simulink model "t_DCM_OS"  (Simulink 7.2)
settings: Solver=ode3  SolverMode=SingleTasking  StartTime=0.0  StopTime=1  FixedStep=10e-6  RelTol=1e-5  AbsTol=1e-6
libraries: simulink x1

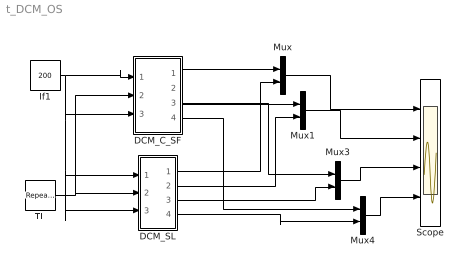
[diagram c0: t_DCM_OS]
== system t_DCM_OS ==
  DCM_C_SF : Subsystem  mask(DCM C-S-Function Block
){Ra=.5, La=3e-3, Rf=200, Lf=1, If0=1, Laf=0.7, J=.0167, D=0.01, W0=0}
      mask prompts: Ra "Armature Resistance"; La "Armature Inductance"; Rf "Field Resistance"; Lf "Filed Inductance"; If0 "Initial field current"; Laf "Mutual Inductance"; J "Moment of Inertia"; D "Damping Coefficient"; W0 "initial ang. speed"
      mask help: Open source D-Motor modeled as Simulink C-S-Function Block Input Vector u: u[0]= Armature Voltage u[1]= Load Torque u[2]= Field Voltage Output Vector y: y[0]= Armature Current y[1]= EMF y[2]= Te y[3]= Ang. Velocity W Parameter Vector p: p[0]= Armature Resistance Ra p[1]= Armature Inductance La p[2]= Field Resistance Rf p[3]= Filed Inductance Lf p[4]= Initial field current ILf0 p[5]= Mutual Ind. Laf p[6]= Moment of Inertia J p[7]= Damp. Coef. D p[8]= Initial Ang. Velocity W0 You can pause the simulation during running, change the Parameters you want and continue the Simulation
  DCM_SL : Subsystem  mask(dcm){Ra=.5, La=3e-3, Rf=200, Lf=1, If0=1, Laf=0.7, J=.0167, D=0.01, omm0=0}
      mask prompts: Ra "Armature Resistance"; La "Armature Inductance"; Rf "Filed Resistance"; Lf "Filed Inductance"; If0 "Initial field current"; Laf "Mutual Inductance"; J "Moment of Inertia"; D "Damping Coefficient"; omm0 "initial ang. speed"
      mask help: Open source D-Motor modeled in Simulink Blocks Input Vector u: u[0]= Armature Voltage u[1]= Load Torque u[2]= Field Voltage Output Vector y: y[0]= Armature Current y[1]= EMF y[2]= Te y[3]= Ang. Velocity W Parameter Vector p: p[0]= Armature Resistance Ra p[1]= Armature Inductance La p[2]= Field Resistance Rf p[3]= Filed Inductance Lf p[4]= Initial field current ILf0 p[5]= Mutual Ind. Laf p[6]= Moment of Inertia J p[7]= Damp. Coef. D p[8]= Initial Ang. Velocity W0 You can pause the simulation during running, change the Parameters you want and continue the Simulation
  If1 : Constant  Value=200
  Mux{,1,3..4} (4 alike) : Mux  Inputs=2
  Scope : Scope  NumInputPorts=4
  TL : simulink/Sources/Repeating Sequence  SystemSampleTime=-1  rep_seq_t="[0   0.2   0.201    0.6    0.601      2 ]"  rep_seq_y="[0     0        40      40      -40      -40]"
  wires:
  DCM_SL/1(ia) -> Mux/2
  DCM_SL/2(emf) -> Mux1/2
  Mux/1 -> Scope/1
  Mux1/1 -> Scope/2
  Mux3/1 -> Scope/3
  DCM_SL/3(Te) -> Mux3/2
  DCM_SL/4(w) -> Mux4/2
  Mux4/1 -> Scope/4
  If1/1 -> DCM_SL/3(Vf), DCM_SL/1(Va), DCM_C_SF/3(vf), DCM_C_SF/1(va)
  TL/1 -> DCM_SL/2(Tl), DCM_C_SF/2(TL)
  DCM_C_SF/1(Ia) -> Mux/1
  DCM_C_SF/2(emf) -> Mux1/1
  DCM_C_SF/3(TE) -> Mux3/1
  DCM_C_SF/4(W) -> Mux4/1

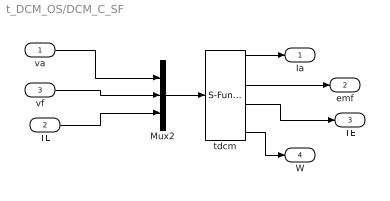
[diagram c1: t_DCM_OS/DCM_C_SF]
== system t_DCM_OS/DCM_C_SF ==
  va : Inport  OutDataType=sfix(16)  OutScaling=2^0
  TL : Inport  Port=2  OutDataType=sfix(16)  OutScaling=2^0
  vf : Inport  Port=3  OutDataType=sfix(16)  OutScaling=2^0
  Mux2 : Mux  Inputs=3
  tdcm : S-Function  FunctionName=s_DCM_OS  Parameters="[Ra La  Rf Lf If0 Laf J D W0]"  EnableBusSupport=off
  Ia : Outport  OutDataType=sfix(16)  OutScaling=2^0
  emf : Outport  Port=2  OutDataType=sfix(16)  OutScaling=2^0
  TE : Outport  Port=3  OutDataType=sfix(16)  OutScaling=2^0
  W : Outport  Port=4  OutDataType=sfix(16)  OutScaling=2^0
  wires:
  Mux2/1 -> tdcm/1
  tdcm/1 -> Ia/1
  va/1 -> Mux2/1
  tdcm/4 -> W/1
  vf/1 -> Mux2/2
  TL/1 -> Mux2/3
  tdcm/2 -> emf/1
  tdcm/3 -> TE/1

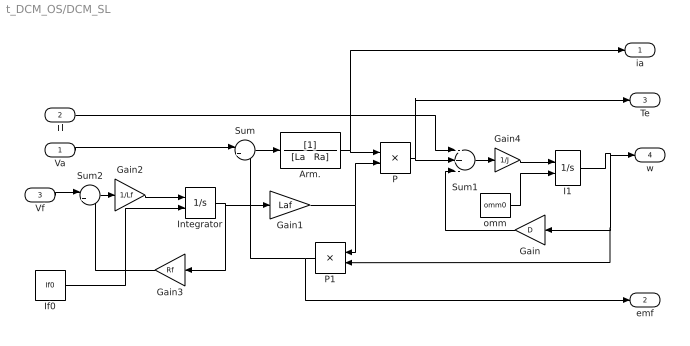
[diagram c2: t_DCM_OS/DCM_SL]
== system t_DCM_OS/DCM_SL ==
  Va : Inport  OutDataType=sfix(16)  OutScaling=2^0
  Tl : Inport  Port=2  OutDataType=sfix(16)  OutScaling=2^0
  Vf : Inport  Port=3  OutDataType=sfix(16)  OutScaling=2^0
  Arm. : TransferFcn  Denominator="[La   Ra]"
  Gain : Gain  Orientation=left  Gain=D  ParameterDataType=sfix(16)  ParameterScaling=2^0  OutDataType=sfix(16)  OutScaling=2^0
  Gain1 : Gain  Gain=Laf  ParameterDataType=sfix(16)  ParameterScaling=2^0  OutDataType=sfix(16)  OutScaling=2^0
  Gain2 : Gain  Gain=1/Lf  ParameterDataType=sfix(16)  ParameterScaling=2^0  OutDataType=sfix(16)  OutScaling=2^0
  Gain3 : Gain  Orientation=left  Gain=Rf  ParameterDataType=sfix(16)  ParameterScaling=2^0  OutDataType=sfix(16)  OutScaling=2^0
  Gain4 : Gain  Gain=1/J  ParameterDataType=sfix(16)  ParameterScaling=2^0  OutDataType=sfix(16)  OutScaling=2^0
  I1 : Integrator  InitialConditionSource=external
  If0 : Constant  Value=If0  OutDataType=sfix(16)  OutScaling=2^0
  Integrator : Integrator  InitialConditionSource=external
  P : Product  OutDataType=sfix(16)  OutScaling=2^0
  P1 : Product  Orientation=left  OutDataType=sfix(16)  OutScaling=2^0
  Sum : Sum  Inputs=|+-  OutDataType=sfix(16)  OutScaling=2^0
  Sum1 : Sum  Inputs=-+-  OutDataType=sfix(16)  OutScaling=2^0
  Sum2 : Sum  Inputs=|+-  OutDataType=sfix(16)  OutScaling=2^0
  omm : Constant  Value=omm0
  ia : Outport
  emf : Outport  Port=2
  Te : Outport  Port=3
  w : Outport  Port=4
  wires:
  I1/1 -> P1/2, Gain/1, w/1
  P1/1 -> emf/1, Sum/2
  P/1 -> Te/1, Sum1/2
  Arm./1 -> ia/1, P/1
  Sum1/1 -> Gain4/1
  Sum/1 -> Arm./1
  Tl/1 -> Sum1/1
  Gain/1 -> Sum1/3
  Va/1 -> Sum/1
  Gain1/1 -> P1/1, P/2
  Vf/1 -> Sum2/1
  Sum2/1 -> Gain2/1
  Integrator/1 -> Gain1/1, Gain3/1
  Gain2/1 -> Integrator/1
  If0/1 -> Integrator/2
  Gain3/1 -> Sum2/2
  Gain4/1 -> I1/1
  omm/1 -> I1/2
